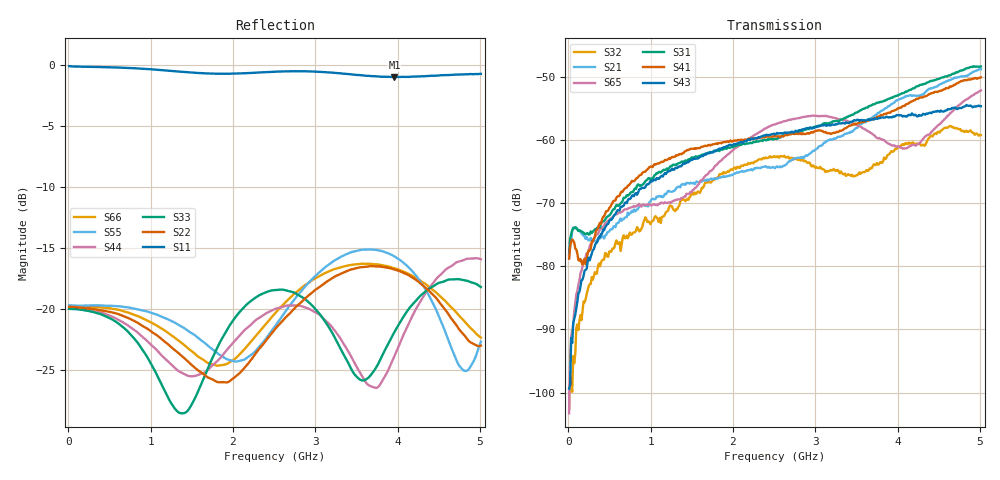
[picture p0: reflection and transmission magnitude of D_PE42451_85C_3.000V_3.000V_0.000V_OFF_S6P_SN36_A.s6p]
! Device ID: PE42451
! Serial: 36
! Insertion: A
! Temp: 85C
! VDD: 3.000
! Control_Hi: 100.000
! Control_Lo: 0.000
! Logic State: OFF
! Port 1: RFC
! Port 2: RF1
! Port 3: RF2
! Port 4: RF3
! Port 5: RF4
! Port 6: RF5
! V1 = 0.00
! V2 = 3.00
! V3 = 3.00
! V4 = 0.00
! IDD: 1.396680e-05
#  Hz  S  RI  R  50
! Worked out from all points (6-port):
!   401 points, 10 MHz to 5.01 GHz, reference 50 ohm
!   strongest paths, dB at 10 MHz, 1.26 GHz, 2.51 GHz, 3.76 GHz, 5.01 GHz:
!     S43: -99.4, -64.5, -59.1, -56.6, -54.6
!     S41: -78.8, -62.7, -59.4, -56.3, -50.1
!     S31: -78.1, -64.1, -59.8, -54.1, -48.4
!     S65: -103.3, -69.7, -57.5, -59.8, -52.1
!     S21: -78.6, -68.2, -64.5, -55.7, -48.8
!     S32: -102.5, -70.5, -62.6, -63.9, -59.2
!   lowest |S11| = -1.0 dB at 3.96 GHz (marker M1), VSWR 17.33, Z = 3.13 - j14.5 ohm
!   |S11| at or under -10 dB: nowhere
